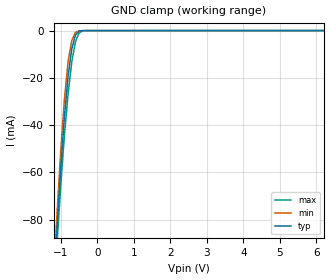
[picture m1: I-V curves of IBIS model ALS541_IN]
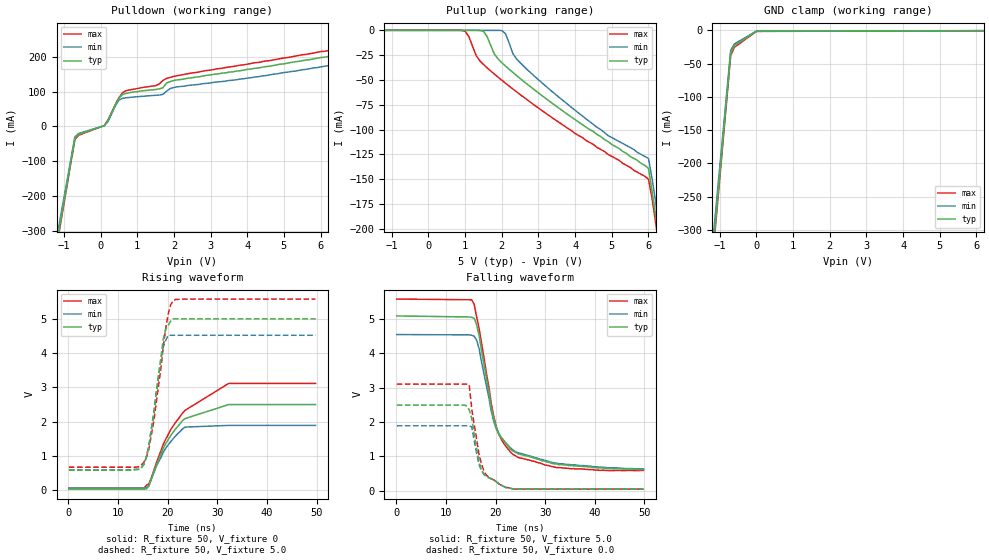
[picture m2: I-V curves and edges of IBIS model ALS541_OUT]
| TEXAS INSTRUMENTS INCORPORATED
| Standard Linear and Logic Group
| IBIS Model of SN74ALS541
| OCTAL BUFFERS AND LINE DRIVERS WITH3-STATE OUTPUTS
| SOIC 20-pin (DW), SOP 20-pin (NS), SSOP 20-pin (DB), P-DIP 20-pin (N) Package
[IBIS Ver]   3.2
[Comment Char]  |_char
[File Name]   sn74als541.ibs
[File Rev]   2.1
[Date]   Sept. 29, 2004
[Source]   Data created from Labo data at TI-SLL.
[Notes]   The following is an IBIS list for the ALS541.
   Please contact sllibis@ti.com with questions and
   comments concerning SLL IBIS models.
   - FILE REV HISTORY
   - 2.1 Re-Release IBIS file on 10/06/04
   - Power clamp data deleted as there is no power-clamp diode.
[Disclaimer] Property of Texas Instruments Incorporated.  Unauthorized
   reproduction and/or distribution is strictly prohibited.
   This product is protected under copyright law.
   Created 2000, (C) Copyright 2000, Texas Instruments Inc.,
   All Rights Reserved.
   UNLESS THERE IS A SIGNED, WRITTEN AGREEMENT TO THE
   CONTRARY, TEXAS INSTRUMENTS () IS PROVIDING THE IBIS
   MODELS  AND WITHOUT ANY WARRANTY, EXPRESSED OR
   IMPLIED.  TI assumes no liability for:
   1) the accuracy of the IBIS models provided to your
   company;
   2) the proper functioning of these IBIS Models in your
   design or for any resulting applications; or
   3) infringement of patents, copyrights or intellectual
   property rights resulting from your use of these IBIS
   models.
   TI provides IBIS Models as a service to our customers.
   You and your company shall not distribute, sell or give
   these models to anyone else without prior written
   permission from TI.
   TI reserves the right to make changes to our products or
   to discontinue any semiconductor product or service
   without notice, and advises our customers to obtain the
   latest version of relevant information to verify, before
   placing orders, that the information being relied on is
   current.
   Please be aware that your receipt and use of the IBIS
   information provided shall serve as acceptance of these
   terms and conditions.  If you do not accept these terms,
   you should return or destroy the IBIS models and any
   other accompanying information immediately.
|   Component ALS541_DW
[Component]   ALS541_DW
[Manufacturer]  Texas Instruments, Inc.
[Package]
|   typ   min   max
R_pkg   0.038   0.033   0.045
L_pkg   5.012nH   4.110nH   6.349nH
C_pkg   0.717pF   0.530pF   0.868pF
[Pin]   signal_name   model_name   R_pin   L_pin   C_pin
1   1OE_NOT   ALS541_IN   0.042   6.336nH   0.865pF
2   A1   ALS541_IN   0.043   5.542nH   0.867pF
3   A2   ALS541_IN   0.034   4.714nH   0.732pF
4   A3   ALS541_IN   0.034   4.377nH   0.591pF
5   A4   ALS541_IN   0.036   4.130nH   0.533pF
6   A5   ALS541_IN   0.035   4.111nH   0.530pF
7   A6   ALS541_IN   0.034   4.284nH   0.583pF
8   A7   ALS541_IN   0.034   4.634nH   0.726pF
9   A8   ALS541_IN   0.040   5.518nH   0.865pF
10   GND   GND   0.043   6.349nH   0.866pF
11   Y8   ALS541_OUT   0.041   6.281nH   0.861pF
12   Y7   ALS541_OUT   0.045   5.561nH   0.868pF
13   Y6   ALS541_OUT   0.033   4.778nH   0.742pF
14   Y5   ALS541_OUT   0.035   4.414nH   0.596pF
15   Y4   ALS541_OUT   0.035   4.110nH   0.533pF
16   Y3   ALS541_OUT   0.036   4.130nH   0.533pF
17   Y2   ALS541_OUT   0.034   4.377nH   0.591pF
18   Y1   ALS541_OUT   0.034   4.714nH   0.731pF
19   2OE_NOT   ALS541_IN   0.043   5.569nH   0.868pF
20   VCC   POWER   0.042   6.308nH   0.864pF
|   Component ALS541_NS
[Component]   ALS541_NS
[Manufacturer]  Texas Instruments, Inc.
[Package]
|   typ   min   max
R_pkg   0.044   0.029   0.058
L_pkg   3.666nH   2.317nH   5.115nH
C_pkg   0.548pF   0.316pF   0.725pF
[Pin]   signal_name   model_name   R_pin   L_pin   C_pin
1   1OE_NOT   ALS541_IN   0.058   5.115nH   0.725pF
2   A1   ALS541_IN   0.053   4.591nH   0.724pF
3   A2   ALS541_IN   0.049   3.754nH   0.572pF
4   A3   ALS541_IN   0.029   2.549nH   0.388pF
5   A4   ALS541_IN   0.031   2.317nH   0.316pF
6   A5   ALS541_IN   0.031   2.317nH   0.316pF
7   A6   ALS541_IN   0.029   2.556nH   0.399pF
8   A7   ALS541_IN   0.049   3.754nH   0.579pF
9   A8   ALS541_IN   0.053   4.591nH   0.724pF
10   GND   GND   0.058   5.115nH   0.725pF
11   Y8   ALS541_OUT   0.058   5.115nH   0.725pF
12   Y7   ALS541_OUT   0.053   4.591nH   0.724pF
13   Y6   ALS541_OUT   0.049   3.754nH   0.579pF
14   Y5   ALS541_OUT   0.029   2.557nH   0.399pF
15   Y4   ALS541_OUT   0.031   2.317nH   0.316pF
16   Y3   ALS541_OUT   0.031   2.317nH   0.316pF
17   Y2   ALS541_OUT   0.029   2.557nH   0.399pF
18   Y1   ALS541_OUT   0.049   3.754nH   0.579pF
19   2OE_NOT   ALS541_IN   0.053   4.591nH   0.724pF
20   VCC   POWER   0.058   5.115nH   0.725pF
|   Component ALS541_DB
[Component]   ALS541_DB
[Manufacturer]  Texas Instruments, Inc.
[Package]
|   typ   min   max
R_pkg   0.040   0.035   0.051
L_pkg   3.495nH   3.035nH   4.314nH
C_pkg   0.420pF   0.346pF   0.502pF
[Pin]   signal_name   model_name   R_pin   L_pin   C_pin
1   1OE_NOT   ALS541_IN   0.049   4.310nH   0.502pF
2   A1   ALS541_IN   0.048   3.903nH   0.487pF
3   A2   ALS541_IN   0.035   3.189nH   0.396pF
4   A3   ALS541_IN   0.035   3.036nH   0.347pF
5   A4   ALS541_IN   0.035   3.035nH   0.367pF
6   A5   ALS541_IN   0.035   3.035nH   0.367pF
7   A6   ALS541_IN   0.035   3.036nH   0.347pF
8   A7   ALS541_IN   0.035   3.189nH   0.397pF
9   A8   ALS541_IN   0.047   3.899nH   0.488pF
10   GND   GND   0.051   4.314nH   0.500pF
11   Y8   ALS541_OUT   0.051   4.314nH   0.500pF
12   Y7   ALS541_OUT   0.047   3.899nH   0.488pF
13   Y6   ALS541_OUT   0.035   3.189nH   0.397pF
14   Y5   ALS541_OUT   0.035   3.036nH   0.346pF
15   Y4   ALS541_OUT   0.035   3.035nH   0.367pF
16   Y3   ALS541_OUT   0.035   3.035nH   0.367pF
17   Y2   ALS541_OUT   0.035   3.036nH   0.346pF
18   Y1   ALS541_OUT   0.035   3.189nH   0.397pF
19   2OE_NOT   ALS541_IN   0.047   3.899nH   0.488pF
20   VCC   POWER   0.051   4.314nH   0.502pF
|   Component ALS541_N
[Component]   ALS541_N
[Manufacturer]  Texas Instruments, Inc.
[Package]
|   Mean.   Min.   Max.
R_pkg   0.043   0.038   0.05
L_pkg   7.384nH   4.68nH   10.321nH
C_pkg   0.51pF   0.231pF   0.821pF
[Pin]   signal_name   model_name   R_pin   L_pin   C_pin
1   1OE_NOT   ALS541_IN   0.042   9.427nH   0.81pF
2   A1   ALS541_IN   0.046   8.544nH   0.456pF
3   A2   ALS541_IN   0.048   7.163nH   0.435pF
4   A3   ALS541_IN   0.04   4.825nH   0.261pF
5   A4   ALS541_IN   0.04   5.284nH   0.648pF
6   A5   ALS541_IN   0.04   4.686nH   0.232pF
7   A6   ALS541_IN   0.04   6.359nH   0.489pF
8   A7   ALS541_IN   0.038   7.982nH   0.475pF
9   A8   ALS541_IN   0.043   9.403nH   0.475pF
10   GND   GND   0.05   10.321nH  0.805pF
11   Y8   ALS541_OUT   0.05   10.281nH  0.81pF
12   Y7   ALS541_OUT   0.043   9.383nH   0.477pF
13   Y6   ALS541_OUT   0.038   7.978nH   0.476pF
14   Y5   ALS541_OUT   0.04   6.302nH   0.492pF
15   Y4   ALS541_OUT   0.04   4.68nH   0.231pF
16   Y3   ALS541_OUT   0.04   5.284nH   0.648pF
17   Y2   ALS541_OUT   0.04   4.822nH   0.261pF
18   Y1   ALS541_OUT   0.047   7.118nH   0.439pF
19   2OE_NOT   ALS541_OUT   0.046   8.492nH   0.461pF
20   VCC   POWER   0.043   9.348nH   0.821pF
| Models and submodels in the file (2): ALS541_IN (Input), ALS541_OUT (3-state)
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|   Model ALS541_IN
[Model]   ALS541_IN
Model_type  Input
Polarity   Non-Inverting
Vinl = 0.8
Vinh = 2.0
| variable   typ   min   max
C_comp   1.33pf   1.00pf   1.66pf
[Temperature Range]   25   0   70
[Voltage Range]   5.0   4.5   5.5
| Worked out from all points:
|   GND clamp passes 1 mA (typ) near -0.55 V on its own axis
[GND Clamp]
|   Voltage   I(typ)   I(min)   I(max)
-5V       -1.26A     -1.34A     -1.17A
-1.2V     -110mA     -105mA     -115mA
-1.1V     -82.6mA    -76.2mA    -89.1mA
-1V       -57.6mA    -50.3mA    -65.1mA
-900mV    -36mA      -28.6mA    -44mA
-800mV    -19.1mA    -13mA      -26.6mA
-700mV    -7.68mA    -4.18mA    -13.2mA
-600mV    -1.94mA    -746uA     -4.77mA
-500mV    -200uA     -48.7uA    -939uA
-400mV    -23.9uA    -19.8uA    -81.2uA
-300mV    -17.3uA    -18.3uA    -18.3uA
10V       590pA      85.9pA     369pA
|   Model ALS541_OUT
[Model]   ALS541_OUT
Model_type  3-state
Polarity   Inverting
Enable   Active-Low
Vmeas = 1.3v
Cref = 0pf
| variable   typ   min   max
C_comp   5.8pf   4.35pf   7.25pf
[Temperature Range]   25   0   70
[Voltage Range]   5.0   4.5   5.5
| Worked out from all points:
|   slope of the pulldown table from 0 to 0.75 V, typ, clamps not added: 7.68 ohm
|   slope of the pullup table from 0 to 0.75 V, typ, clamps not added: 61.6 kohm
|   rising waveform, R_fixture 50, V_fixture 0: 20-80 % time 5.65ns typ, 4.25ns min, 8.04ns max; typ from 0.022 V to 2.5 V
|   falling waveform, R_fixture 50, V_fixture 5.0: 20-80 % time 4.3ns typ, 4.79ns min, 3.98ns max; typ from 5.08 V to 0.625 V
|   rising waveform, R_fixture 50, V_fixture 5.0: 20-80 % time 2.44ns typ, 2.3ns min, 2.73ns max; typ from 0.583 V to 5.01 V
|   falling waveform, R_fixture 50, V_fixture 0.0: 20-80 % time 2.13ns typ, 2.55ns min, 2.33ns max; typ from 2.49 V to 0.05 V
[Pulldown]
|   Voltage   I(typ)   I(min)   I(max)
-5V       -2.66A     -2.56A     -2.7A
-1.2V     -339mA     -324mA     -348mA
-1.1V     -278mA     -265mA     -286mA
-700mV    -34mA      -30mA      -38mA
-600mV    -22.8mA    -20.4mA    -25.6mA
100mV     2.18mA     2mA        2.4mA
500mV     80.8mA     75.4mA     82.6mA
600mV     91.9mA     80.8mA     96.9mA
1.5V      106mA      89.5mA     117mA
1.7V      111mA      92.1mA     132mA
2V        132mA      112mA      144mA
10V       266mA      237mA      287mA
[Pullup]
|   Voltage   I(typ)   I(min)   I(max)
-5V       17.2uA     5.77uA     28.9uA
900mV     21.3nA     205pA      -48.7uA
1.1V      21.3nA     205pA      -6.17mA
1.5V      -956uA     205pA      -34.3mA
2V        -32.5mA    -169uA     -50.2mA
2.4V      -45.4mA    -28.6mA    -61.8mA
3V        -63mA      -49.8mA    -78.2mA
4.9V      -112mA     -106mA     -125mA
6V        -139mA     -129mA     -150mA
6.2V      -187mA     -174mA     -195mA
6.3V      -212mA     -198mA     -220mA
10V       -1.11A     -1.09A     -1.15A
[GND Clamp]
|   Voltage   I(typ)   I(min)   I(max)
-5V       -2.66A     -2.56A     -2.7A
-1.2V     -339mA     -324mA     -348mA
-1.1V     -278mA     -265mA     -286mA
-700mV    -34mA      -30mA      -38mA
-600mV    -22.8mA    -20.4mA    -25.6mA
0V        -1.4mA     -1.2mA     -1.6mA
10V       1.4uA      1.2uA      1.6uA
[Ramp]
| variable   typ   min   max
dV/dt_r   1.478/5.728n   1.284/5.643n   1.662/6.137n
dV/dt_f   2.724/4.371n   2.424/5.041n   2.874/4.019n
R_load = 50
[Rising Waveform]
R_fixture = 50
V_fixture = 0
|   Time   V(typ)   V(min)   V(max)
97.7ps    22.3mV     50.6mV     53.1mV
15.2ns    22.3mV     50.6mV     53.1mV
16.2ns    105mV      115mV      179mV
17.7ns    717mV      683mV      786mV
19.6ns    1.35V      1.22V      1.48V
20.6ns    1.59V      1.41V      1.76V
23ns      2.03V      1.79V      2.25V
23.5ns    2.09V      1.84V      2.33V
32.3ns    2.5V       1.89V      3.12V
49.8ns    2.5V       1.89V      3.12V
[Falling Waveform]
R_fixture = 50
V_fixture = 5.0
V_fixture_min = 4.5
V_fixture_max = 5.5
|   Time   V(typ)   V(min)   V(max)
97.7ps    5.08V      4.54V      5.57V
15.2ns    5.04V      4.52V      5.55V
15.7ns    5.01V      4.49V      5.41V
16.7ns    4.5V       4.12V      4.71V
19.1ns    2.44V      2.33V      2.56V
20.1ns    1.86V      1.81V      1.89V
21.1ns    1.56V      1.56V      1.51V
23.5ns    1.16V      1.19V      1.06V
32.3ns    781mV      808mV      677mV
49.8ns    625mV      635mV      596mV
[Rising Waveform]
R_fixture = 50
V_fixture = 5.0
V_fixture_min = 4.5
V_fixture_max = 5.5
|   Time   V(typ)   V(min)   V(max)
97.7ps    583mV      581mV      665mV
12.8ns    583mV      581mV      665mV
15.2ns    754mV      744mV      805mV
16.2ns    1.26V      1.3V       1.19V
17.2ns    2.23V      2.25V      2.01V
18.2ns    3.41V      3.38V      3.1V
19.1ns    4.41V      4.18V      4.18V
20.1ns    4.82V      4.53V      5.15V
21.1ns    5.01V      4.53V      5.54V
49.8ns    5.01V      4.53V      5.59V
[Falling Waveform]
R_fixture = 50
V_fixture = 0.0
|   Time   V(typ)   V(min)   V(max)
97.7ps    2.49V      1.89V      3.1V
13.8ns    2.49V      1.89V      3.1V
14.7ns    2.35V      1.89V      3.07V
15.2ns    2.11V      1.86V      2.38V
15.7ns    1.63V      1.45V      1.92V
16.7ns    818mV      744mV      1.03V
17.7ns    476mV      473mV      551mV
18.7ns    376mV      376mV      393mV
22.1ns    97.5mV     97.7mV     97.9mV
49.8ns    50.5mV     51.2mV     50mV
